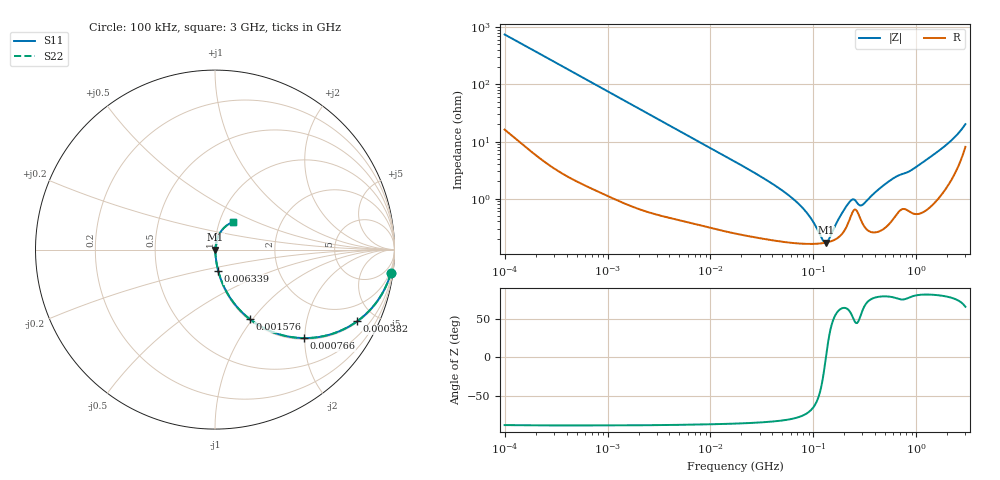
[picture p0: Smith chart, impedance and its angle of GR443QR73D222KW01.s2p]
!Murata Part Number: GR443QR73D222KW01
!These Parameters are Measured in Series Mode Connection
!Data Generated on Mar 13, 2026
!  o--ll--o
!Port1  Port2
!  o------o
!Operation Temp=25[degC], DC Bias Voltage=0[V]
!Freq. Start=100[kHz] Stop=3[GHz] 401[Steps]
# Hz S RI R 50
!Freq.(Hz) S11(Real) S11(Imag) S21(Real) S21(Imag) S12(Real) S12(Imag) S22(Real) S22(Imag)
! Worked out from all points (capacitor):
!   401 points, 100 kHz to 3 GHz, reference 50 ohm
!   read as one part in series: C = 2.13 nF near 105.3 kHz
!   lowest |Z| = 170 mohm at 132.7 MHz (marker M1)
!   series resonance near 132.3 MHz, so ESL is about 680 pH
!   S11 on the Smith chart (normalised r, x): 100 kHz: 1, -15; 382 kHz: 1.05, -3.95; 766 kHz: 1.03, -1.98; 1.576 MHz: 1.02, -0.97; 6.339 MHz: 1.01, -0.24; 3 GHz: 1.16, +0.37
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100000  0.9796 -0.131  0.0204 0.131  0.0204 0.131  0.9796 -0.131
216663  0.9199 -0.264  0.0801 0.264  0.0801 0.264  0.9199 -0.264
381967  0.7925 -0.3989  0.2075 0.3989  0.2075 0.3989  0.7925 -0.3989
562235  0.6417 -0.4728  0.3583 0.4728  0.3583 0.4728  0.6417 -0.4728
766005  0.4941 -0.493  0.5059 0.493  0.5059 0.493  0.4941 -0.493
1576268  0.1929 -0.3866  0.8071 0.3866  0.8071 0.3866  0.1929 -0.3866
3161081  0.0595 -0.2262  0.9405 0.2262  0.9405 0.2262  0.0595 -0.2262
6339300  0.0181 -0.1186  0.9819 0.1186  0.9819 0.1186  0.0181 -0.1186
1.77727e7  0.00428 -0.043  0.9957 0.043  0.9957 0.043  0.00428 -0.043
5.523785e7  0.00186 -0.012  0.9981 0.012  0.9981 0.012  0.00186 -0.012
7.722238e7  0.00168 -0.00693  0.9983 0.00693  0.9983 0.00693  0.00168 -0.00693
9.738194e7  0.00163 -0.00386  0.9984 0.00386  0.9984 0.00386  0.00163 -0.00386
1.228043e8  0.00166 -0.000945  0.9983 0.000945  0.9983 0.000945  0.00166 -0.000945
1.326759e8  0.0017 3.19e-05  0.9983 -3.19e-05  0.9983 -3.19e-05  0.0017 3.19e-05
1.90323e8  0.00245 0.00507  0.9975 -0.00507  0.9975 -0.00507  0.00245 0.00507
2.279507e8  0.00463 0.00771  0.9954 -0.00771  0.9954 -0.00771  0.00463 0.00771
2.462744e8  0.00626 0.00736  0.9937 -0.00736  0.9937 -0.00736  0.00626 0.00736
3.026647e8  0.00363 0.00697  0.9964 -0.00697  0.9964 -0.00697  0.00363 0.00697
5.475153e8  0.00402 0.0199  0.996 -0.0199  0.996 -0.0199  0.00402 0.0199
8.706963e8  0.00669 0.0297  0.9933 -0.0297  0.9933 -0.0297  0.00669 0.0297
1.384641e9  0.0101 0.053  0.9899 -0.053  0.9899 -0.053  0.0101 0.053
3e9  0.1007 0.1534  0.8993 -0.1534  0.8993 -0.1534  0.1007 0.1534
